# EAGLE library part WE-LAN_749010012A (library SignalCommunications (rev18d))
LAN-Transformer WE-LAN 10/100 Base T - Compliant with IEEE 802.3 standards - SMD -- Ethernet -- Power over Ethernet -- 1 Gigabit Ethernet -- Compliant with most IC's for ethernet applications like Intel, AMD, Globespan and Realtek -- Hub, Router, Switch Details see: http://katalog.we-online.de/en/pbs/WE-LAN/S/749010012A? 2016 (C) Würth Elektronik
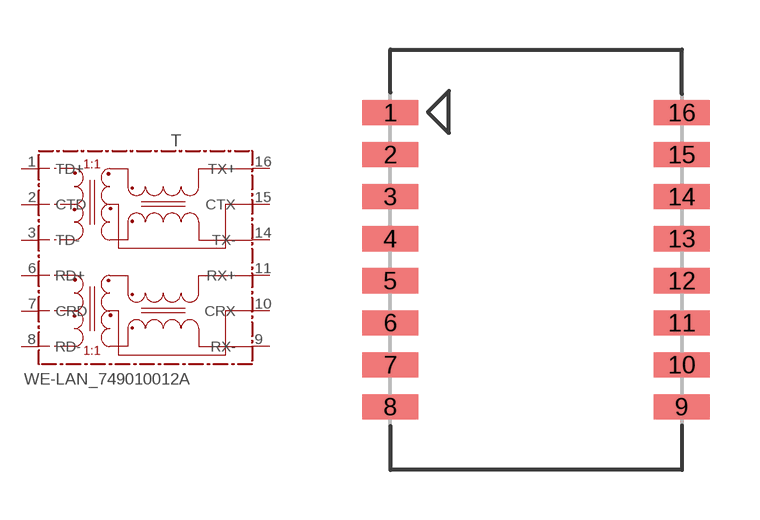
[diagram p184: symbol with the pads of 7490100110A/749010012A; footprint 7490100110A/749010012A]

Designator prefix T

## WE-LAN_749010012A  [7490100110A/749010012A]
1  TD+
2  CTD
3  TD-
6  RD+
7  CRD
8  RD-
9  RX-
10  CRX
11  RX+
14  TX-
15  CTX
16  TX+

## Footprint 7490100110A/749010012A (pad centres in mm)
smd 1.7 x 0.76: 1 -4.4,4.445; 2 -4.4,3.175; 3 -4.4,1.905; 4 -4.4,0.635; 5 -4.4,-0.635; 6 -4.4,-1.905; 7 -4.4,-3.175; 8 -4.4,-4.445; 9 4.4,-4.445; 10 4.4,-3.175; 11 4.4,-1.905; 12 4.4,-0.635; 13 4.4,0.635; 14 4.4,1.905; 15 4.4,3.175; 16 4.4,4.445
